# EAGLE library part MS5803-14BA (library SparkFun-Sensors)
Measurement Specialties MS5803_14BA Pressure (Depth) Sensor The MS5803-14BA is a new generation of high resolution pressure sensors with SPI and I2C bus interface. It is optimized for depth measurement systems with a water depth resolution of 1cm and below. The sensor module includes a high linear pressure sensor and an ultra low power 24 bit ΔΣ ADC with internal factory calibrated coefficients. It provides a precise digital 24 Bit pressure and temperature value and different operation modes that allow the user to optimize for conversion speed and current consumption. Datasheet SparkFun Products SparkFun Pressure Sensor Breakout - MS5803-14BA (SEN-12909)
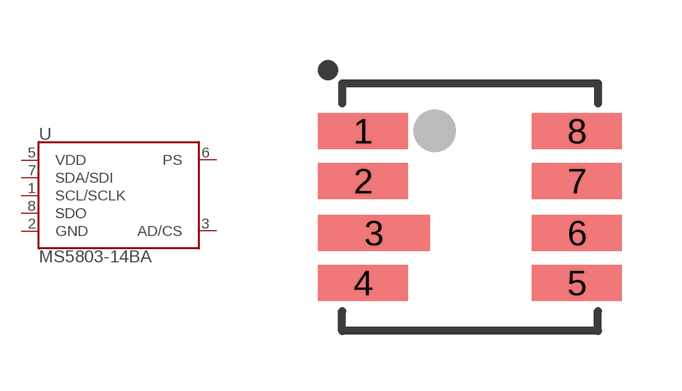
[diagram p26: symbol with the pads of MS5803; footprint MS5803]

Designator prefix U

## MS5803-14BA (PROD_ID: IC-12111)  [MS5803]
1  SCL/SCLK
2  GND
3  AD/CS
5  VDD
6  PS
7  SDA/SDI
8  SDO

## Footprint MS5803 (pad centres in mm)
MS5803-14BA Pressure Sensor 8-Pin 6.4 x6.2 mm Datasheet Specifications: Pin Count: 8 Dimensions: 6.4 x 6.2 x 2.88 mm Pitch: 1.25 mm Devices Using: MS5803-14BA
smd 2.25 x 0.9: 1 -2.675,1.9; 2 -2.675,0.65; 4 -2.675,-1.9; 5 2.675,-1.9; 6 2.675,-0.65; 7 2.675,0.65; 8 2.675,1.9
smd 2.8 x 0.9: 3 -2.4,-0.65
